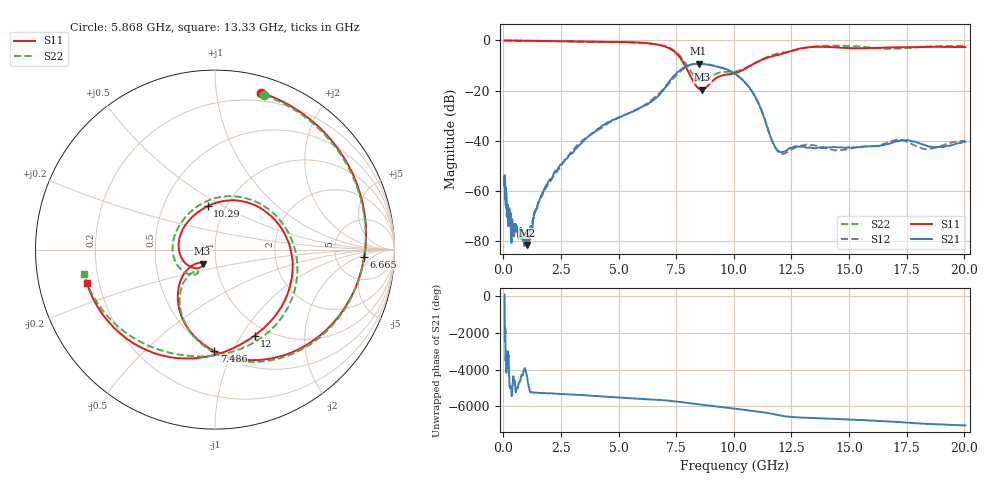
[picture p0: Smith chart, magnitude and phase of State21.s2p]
# Hz S DB R 50
!freq MagS11 AngS11 MagS21 AngS21 MagS12 AngS12 MagS22 AngS22
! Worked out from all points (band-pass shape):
!   1601 points, 50 MHz to 20.05 GHz, reference 50 ohm
!   highest |S21| = -9.20 dB at 8.471 GHz (marker M1); lowest = -81.5 dB at 1.036 GHz (marker M2)
!   |S21| within 3 dB of the highest: 7.625 GHz to 9.851 GHz (2.226 GHz wide, 25.5 % of centre)
!   lowest |S11| = -19.6 dB at 8.631 GHz (marker M3), VSWR 1.23, Z = 43 - j6.86 ohm
!   |S11| at or under -10 dB: 7.879 GHz to 10.72 GHz (2.841 GHz wide, 30.6 % of centre)
!   |S22| runs from -16.2 to 0.0 dB; largest |S21 - S12| = 0.021
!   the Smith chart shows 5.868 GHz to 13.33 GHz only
!   S11 on the Smith chart (normalised r, x): 5.868 GHz: 0.13, +1.33; 6.665 GHz: 10, -3; 7.486 GHz: 0.51, -0.85; 10.29 GHz: 0.82, +0.42; 12 GHz: 0.86, -1.14; 13.33 GHz: 0.15, -0.13
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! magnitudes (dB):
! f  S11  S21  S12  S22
! 50 MHz  0.0  -58.2  -54.2  0.0
! 60.07 MHz  0.0  -55.1  -55.8  0.0
! 100.4 MHz  0.0  -64.2  -63.2  0.0
! 110.6 MHz  0.0  -60.6  -66.4  0.0
! 135.9 MHz  0.0  -65.7  -66.5  0.0
! 209.9 MHz  0.0  -72.6  -73.5  0.0
! 305.3 MHz  0.0  -68.9  -72.2  0.0
! 342.9 MHz  0.0  -79.9  -73.9  0.0
! 369.6 MHz  0.0  -73.7  -72.2  0.0
! 1.005 GHz  -0.1  -79.4  -79.4  -0.1
! 1.036 GHz  -0.1  -81.5  -79.0  -0.1
! 2.722 GHz  -0.3  -47.3  -47.1  -0.4
! 5.868 GHz  -0.8  -27.1  -27.2  -0.9
! 6.665 GHz  -1.6  -22.6  -21.8  -1.6
! 7.402 GHz  -4.3  -14.1  -14.9  -4.0
! 7.486 GHz  -5.0  -13.3  -14.0  -4.6
! 8.471 GHz  -19.1  -9.2  -9.2  -15.9
! 8.631 GHz  -19.6  -9.4  -9.2  -16.2
! 10.29 GHz  -12.2  -15.0  -15.0  -11.8
! 12 GHz  -5.6  -44.4  -45.0  -5.0
! 13.33 GHz  -2.6  -42.7  -41.6  -2.6
! 20.05 GHz  -2.6  -40.4  -40.0  -2.2
